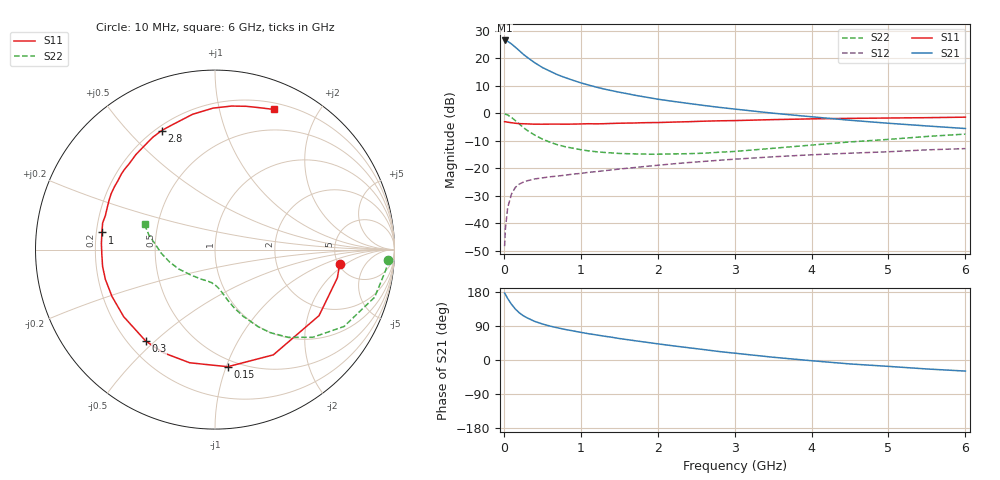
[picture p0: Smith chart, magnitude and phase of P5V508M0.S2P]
! SIEMENS Small Signal Semiconductors
! BFP183
! Si NPN RF Bipolar Junction Transistor in SOT143
! VCE = 0.5 V  IC = 8 mA
! Common Emitter S-Parameters:  March  1996
# GHz  S  MA  R  50
!  f  S11  S21  S12  S22
! GHz  MAG  ANG  MAG  ANG  MAG  ANG  MAG  ANG
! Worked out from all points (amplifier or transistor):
!   36 points, 10 MHz to 6 GHz, reference 50 ohm
!   highest |S21| = 26.5 dB at 10 MHz (marker M1)
!   |S21| within 3 dB of that: start of sweep to 171.8 MHz
!   unconditionally stable (mu >= 1): 996.8 MHz to end of sweep
!   at 250 MHz: K = 0.33, MSG = 23.3 dB, |S12| = -25.1 dB
!   at 1.4 GHz: K = 1.17, MAG = 11.9 dB, |S12| = -20.6 dB
!   at 6 GHz: K = 1.15, MAG = 1.3 dB, |S12| = -12.9 dB
!   S11 on the Smith chart (normalised r, x): 10 MHz: 5.13, -1.62; 150 MHz: 0.44, -1.01; 300 MHz: 0.27, -0.47; 1 GHz: 0.22, +0.07; 2.8 GHz: 0.22, +0.63; 6 GHz: 0.27, +1.47
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0.01  0.6996 -6.6  21.09 176.6  0.0038 82.9  0.9672 -3.3
0.02  0.6997 -13.0  20.97 173.2  0.0078 84.3  0.9584 -6.8
0.05  0.6865 -32.4  20.34 162.2  0.0192 75.6  0.9282 -16.6
0.1  0.6705 -61.0  18.21 146.8  0.0339 61.5  0.8367 -30.8
0.15  0.6564 -83.8  15.88 134.4  0.0447 52.3  0.7316 -41.9
0.2  0.6461 -102.6  13.79 124.7  0.0511 45.9  0.6371 -50.1
0.25  0.6427 -116.5  11.91 117.2  0.0554 40.7  0.5552 -56.4
0.3  0.6392 -127.1  10.49 111.5  0.0587 38.1  0.4902 -60.9
0.4  0.6313 -143.7  8.322 102.0  0.0636 34.1  0.4008 -67.3
0.5  0.6305 -155.5  6.803 95.1  0.0665 31.9  0.3393 -71.9
0.6  0.6329 -164.8  5.814 89.5  0.0696 31.3  0.2962 -75.4
0.7  0.6333 -171.5  5 84.8  0.0719 31.3  0.2658 -78.1
0.8  0.6311 -177.8  4.433 80.5  0.0745 31.5  0.2451 -80.3
1  0.6373 171.4  3.566 73.0  0.0801 31.9  0.2166 -84.6
1.1  0.6434 166.7  3.26 69.4  0.0839 32.2  0.2063 -87.0
1.5  0.6571 151.7  2.41 56.7  0.0961 33.2  0.1851 -95.8
2.2  0.6888 129.8  1.643 37.4  0.1197 31.9  0.1814 -114.2
2.8  0.7269 114.1  1.278 22.3  0.1392 28.9  0.1948 -132.3
3.5  0.7642 99.4  1 7.3  0.1609 24.5  0.2298 -152.1
4.5  0.8051 83.4  0.744 -10.4  0.1871 16.8  0.3001 -176.1
5.5  0.8291 72.4  0.586 -23.7  0.2152 10.0  0.3774 167.5
6  0.847 67.2  0.526 -29.2  0.2268 5.6  0.4167 160.3
